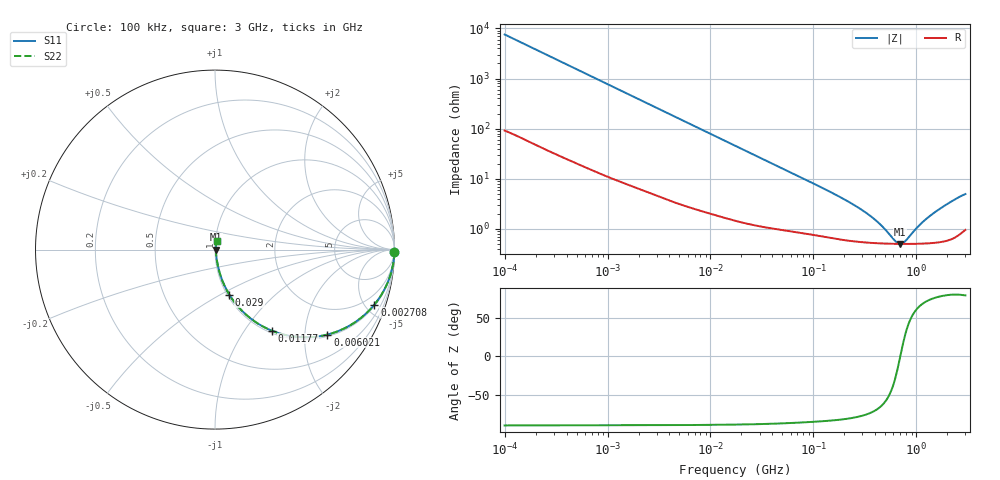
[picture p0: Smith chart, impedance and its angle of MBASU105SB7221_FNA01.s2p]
! MBASU105SB7221_FNA01  S-PARAMETER MODEL  ( Standard Model )
! Model Generated by TAIYO YUDEN Corporation (http://www.ty-top.com)
! Version 1.0
! TAIYO YUDEN Control No. 220601
! Copyright(c) 2017 TAIYO YUDEN CO.,LTD. All Rights Reserved.
! Product Description (link to TY-COMPAS)
! https://ds.yuden.co.jp/TYCOMPAS/or/detail?pn=MBASU105SB7221KFNA01&u=M
! Products Name : Multilayer Ceramic Capacitors
! Characteristics :
!  Capacitance : 220 [pF] , Rated Voltage : 50 [V] , TCC : X7R
!  Case Size : 1.0 x 0.5 / 0.039 x 0.02 [mm/inch] , Thickness : 0.5 / 0.02 [mm/inch]
!  (Conditions: Temperature = 25 [degC] , DC Bias Voltage = 0 [V])
! External Node Assignments :
!  1  o---| |---o  2
! GND o---------o GND
! Frequency Range : 100kHz  -  3GHz  [ 401 STEP ]
# MHZ S RI R 50
! Freq[MHz].  S11 Real  S11 Imag  S21 Real  S21 Imag  S12 Real  S12 Imag  S22 Real  S22 Imag
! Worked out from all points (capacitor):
!   401 points, 100 kHz to 3 GHz, reference 50 ohm
!   read as one part in series: C = 210 pF near 105.3 kHz
!   lowest |Z| = 504 mohm at 690.4 MHz (marker M1)
!   series resonance near 698.8 MHz, so ESL is about 250 pH
!   S11 on the Smith chart (normalised r, x): 100 kHz: open; 2.708 MHz: 1.10, -5.75; 6.021 MHz: 1.06, -2.61; 11.77 MHz: 1.04, -1.34; 29 MHz: 1.02, -0.55; 3 GHz: 1.02, +0.10
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0.1  0.9997 -0.0132  0.000335 0.0132  0.000335 0.0132  0.9997 -0.0132
0.562235  0.9937 -0.0727  0.00629 0.0727  0.00629 0.0727  0.9937 -0.0727
1.282589  0.9709 -0.1607  0.0291 0.1607  0.0291 0.1607  0.9709 -0.1607
2.708188  0.8879 -0.307  0.1121 0.307  0.1121 0.307  0.8879 -0.307
3.161081  0.8544 -0.3439  0.1456 0.3439  0.1456 0.3439  0.8544 -0.3439
6.020821  0.6268 -0.4732  0.3732 0.4732  0.3732 0.4732  0.6268 -0.4732
8.417093  0.4675 -0.4872  0.5325 0.4872  0.5325 0.4872  0.4675 -0.4872
11.76708  0.3156 -0.4514  0.6844 0.4514  0.6844 0.4514  0.3156 -0.4514
17.7727  0.1743 -0.3636  0.8257 0.3636  0.8257 0.3636  0.1743 -0.3636
29.00125  0.0794 -0.2504  0.9206 0.2504  0.9206 0.2504  0.0794 -0.2504
51.12795  0.0327 -0.1503  0.9673 0.1503  0.9673 0.1503  0.0327 -0.1503
97.38194  0.0142 -0.0808  0.9858 0.0808  0.9858 0.0808  0.0142 -0.0808
294.964  0.00596 -0.0232  0.994 0.0232  0.994 0.0232  0.00596 -0.0232
412.3589  0.00534 -0.0132  0.9947 0.0132  0.9947 0.0132  0.00534 -0.0132
547.5153  0.00508 -0.00591  0.9949 0.00591  0.9949 0.00591  0.00508 -0.00591
639.0768  0.00502 -0.00215  0.995 0.00215  0.995 0.00215  0.00502 -0.00215
690.4488  0.005 -0.000286  0.995 0.000286  0.995 0.000286  0.005 -0.000286
785.4083  0.00501 0.00282  0.995 -0.00282  0.995 -0.00282  0.00501 0.00282
1070.062  0.00515 0.0106  0.9948 -0.0106  0.9948 -0.0106  0.00515 0.0106
1420.79  0.00554 0.0186  0.9945 -0.0186  0.9945 -0.0186  0.00554 0.0186
2201.951  0.0074 0.0344  0.9926 -0.0344  0.9926 -0.0344  0.0074 0.0344
3000  0.0118 0.0477  0.9882 -0.0477  0.9882 -0.0477  0.0118 0.0477
